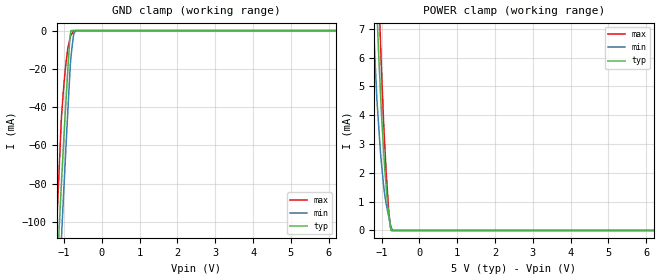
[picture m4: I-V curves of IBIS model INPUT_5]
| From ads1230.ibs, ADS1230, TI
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|   Input INPUT 5V Model
[Model] INPUT_5
Model_type Input
| Signals   GAIN(4), SPEED(13), _PWDN(14), SCLK(15)
Vinl = 1
Vinh = 3.5
|   typ   min   max
|   (nom PVT)   (Fast PVT)   (slow PVT)
|Average
C_comp   8.707e-13   8.645e-13   8.918e-13
| Where   nom PVT is  Nominal Process, 5.0V, 25C
|   Fast PVT is Strong Process, 5.25V, -40C
|   Slow PVT is Weak Process, 4.75V, 85C
[model spec]
Vinl   1   0.95   1.05
Vinh   3.5   3.325   3.675
[Voltage Range]   5   4.75   5.25
|Ambient Temperature   25   85   -40
|Junction Temperature
[Temperature Range]   25   85   -40
[Power Clamp Reference]   5   4.75   5.25
[GND Clamp Reference]   0   0   0
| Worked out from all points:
|   GND clamp passes 1 mA (typ) near -0.83 V on its own axis
|   POWER clamp passes 1 mA (typ) near -0.85 V on its own axis
[GND Clamp]
|   Voltage   I(typ)   I(min)   I(max)
-5V       -2.009A    -2.035A    -1.986A
-1.294V   -178.2mA   -209.4mA   -146mA
-1.155V   -113.5mA   -145.3mA   -83.53mA
-1.138V   -106.7mA   -137.6mA   -75.98mA
-1.062V   -77.14mA   -105.7mA   -43.35mA
-989mV    -50.06mA   -76.07mA   -24.62mA
-947mV    -35.83mA   -59.52mA   -16.39mA
-850mV    -4.763mA   -23.29mA   -4.76mA
-815.7mV  0A         -13.62mA   -2.212mA
-744mV    0A         -1.619mA   0A
-691.7mV  0A         0A         0A
10V       0A         0A         0A
[POWER Clamp]
|   Voltage   I(typ)   I(min)   I(max)
-5V       202.5mA    169.6mA    248.6mA
-1.252V   13mA       8.28mA     18.08mA
-1.176V   9.655mA    5.991mA    13.93mA
-1.119V   7.48mA     4.451mA    10.79mA
-1.062V   5.699mA    3.347mA    7.808mA
-1.034V   4.906mA    2.788mA    6.72mA
-947mV    2.817mA    1.568mA    3.785mA
-915mV    2.122mA    1.225mA    2.944mA
-878.8mV  1.521mA    923.1uA    2.011mA
-815.7mV  611.1uA    511.5uA    772.9uA
-745mV    0A         109.5uA    0A
10V       0A         0A         0A
